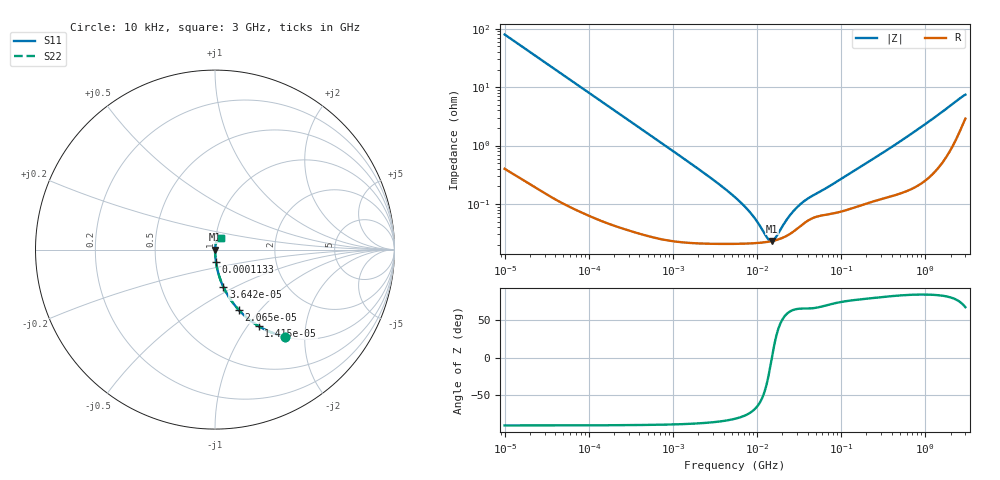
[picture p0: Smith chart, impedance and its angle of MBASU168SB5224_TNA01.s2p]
! MBASU168SB5224_TNA01  S-PARAMETER MODEL  ( Standard Model )
! Model Generated by TAIYO YUDEN Corporation (http://www.ty-top.com)
! Version 3.0
! TAIYO YUDEN Control No. 240510
! Copyright(c) 2012 TAIYO YUDEN CO.,LTD. All Rights Reserved.
! Product Description (link to TY-COMPAS)
! https://ds.yuden.co.jp/TYCOMPAS/or/detail?pn=MBASU168SB5224KTNA01&u=M
! Products Name : Multilayer Ceramic Capacitors
! Characteristics :
!  Capacitance : 0.22 [uF] , Rated Voltage : 50 [V] , TCC : X5R
!  Case Size : 1.6 x 0.8 / 0.063 x 0.031 [mm/inch] , Thickness : 0.8 / 0.031 [mm/inch]
!  (Conditions: Temperature = 25 [degC] , DC Bias Voltage = 0 [V])
! External Node Assignments :
!  1  o---| |---o  2
! GND o---------o GND
! Frequency Range : 10kHz  -  3GHz  [ 401 STEP ]
# MHZ S RI R 50
! Freq[MHz].  S11 Real  S11 Imag  S21 Real  S21 Imag  S12 Real  S12 Imag  S22 Real  S22 Imag
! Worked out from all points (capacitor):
!   401 points, 10 kHz to 3 GHz, reference 50 ohm
!   read as one part in series: C = 199 nF near 10.65 kHz
!   lowest |Z| = 23.1 mohm at 15.02 MHz (marker M1)
!   series resonance near 15.02 MHz, so ESL is about 560 pH
!   S11 on the Smith chart (normalised r, x): 10 kHz: 1.01, -1.60; 14.15 kHz: 1.01, -1.13; 20.65 kHz: 1.00, -0.78; 36.42 kHz: 1.00, -0.44; 113.3 kHz: 1.00, -0.14; 3 GHz: 1.06, +0.14
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0.01  0.3899 -0.4852  0.6101 0.4852  0.6101 0.4852  0.3899 -0.4852
0.014146  0.2432 -0.4264  0.7568 0.4264  0.7568 0.4264  0.2432 -0.4264
0.020651  0.132 -0.3357  0.868 0.3357  0.868 0.3357  0.132 -0.3357
0.036425  0.0473 -0.2094  0.9527 0.2094  0.9527 0.2094  0.0473 -0.2094
0.082683  0.0101 -0.0962  0.9899 0.0962  0.9899 0.0962  0.0101 -0.0962
0.11333  0.00559 -0.0706  0.9944 0.0706  0.9944 0.0706  0.00559 -0.0706
0.683653  0.000393 -0.0118  0.9996 0.0118  0.9996 0.0118  0.000393 -0.0118
2.652321  0.000217 -0.00297  0.9998 0.00297  0.9998 0.00297  0.000217 -0.00297
5.477226  0.000209 -0.00129  0.9998 0.00129  0.9998 0.00129  0.000209 -0.00129
8.252149  0.000211 -0.00069  0.9998 0.00069  0.9998 0.00069  0.000211 -0.00069
9.97066  0.000214 -0.000458  0.9998 0.000458  0.9998 0.000458  0.000214 -0.000458
13.24217  0.000224 -0.000138  0.9998 0.000138  0.9998 0.000138  0.000224 -0.000138
14.10408  0.000227 -6.87e-05  0.9998 6.87e-05  0.9998 6.87e-05  0.000227 -6.87e-05
15.02209  0.000231 2.29e-07  0.9998 -2.29e-07  0.9998 -2.29e-07  0.000231 2.29e-07
16.51234  0.000239 0.000104  0.9998 -0.000104  0.9998 -0.000104  0.000239 0.000104
21.93027  0.000278 0.000424  0.9997 -0.000424  0.9997 -0.000424  0.000278 0.000424
27.34599  0.00034 0.000685  0.9997 -0.000685  0.9997 -0.000685  0.00034 0.000685
34.09912  0.000436 0.000944  0.9996 -0.000944  0.9996 -0.000944  0.000436 0.000944
45.28751  0.000568 0.00125  0.9994 -0.00125  0.9994 -0.00125  0.000568 0.00125
374.4521  0.0014 0.00878  0.9986 -0.00878  0.9986 -0.00878  0.0014 0.00878
1648.003  0.00686 0.0384  0.9931 -0.0384  0.9931 -0.0384  0.00686 0.0384
3000  0.0324 0.0644  0.9676 -0.0644  0.9676 -0.0644  0.0324 0.0644
